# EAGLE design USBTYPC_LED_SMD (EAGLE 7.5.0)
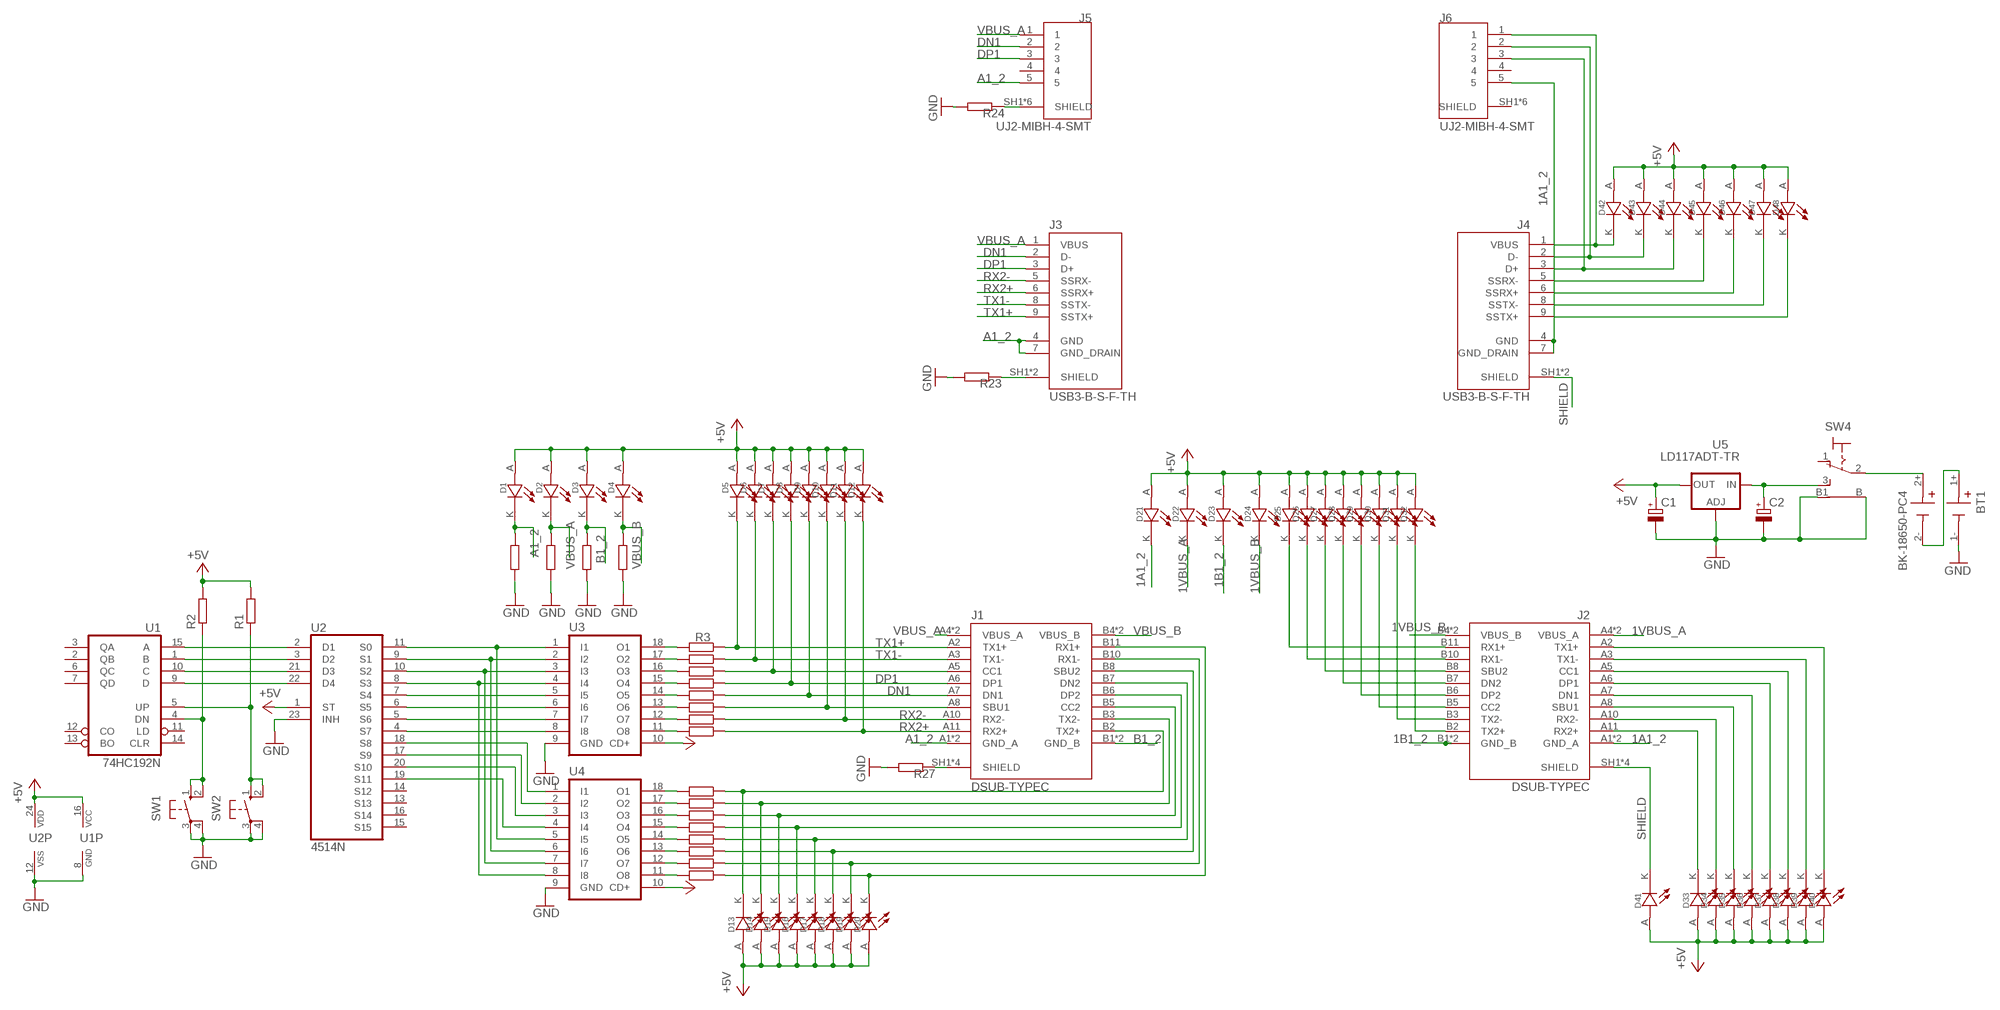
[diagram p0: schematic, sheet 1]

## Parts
BT1  BK-18650-PC4  [BAT_BK-18650-PC4]
C1  CPOL-EUSMCD  [SMC_D]
C2  CPOL-EUSMCD  [SMC_D]
D1  597-6401-607F  [LED_597-6401-607F]
D2  597-6401-607F  [LED_597-6401-607F]
D3  597-6401-607F  [LED_597-6401-607F]
D4  597-6401-607F  [LED_597-6401-607F]
D5  597-6401-607F  [LED_597-6401-607F]
D6  597-6401-607F  [LED_597-6401-607F]
D7  597-6401-607F  [LED_597-6401-607F]
D8  597-6401-607F  [LED_597-6401-607F]
D9  597-6401-607F  [LED_597-6401-607F]
D10  597-6401-607F  [LED_597-6401-607F]
D11  597-6401-607F  [LED_597-6401-607F]
D12  597-6401-607F  [LED_597-6401-607F]
D13  597-6401-607F  [LED_597-6401-607F]
D14  597-6401-607F  [LED_597-6401-607F]
D15  597-6401-607F  [LED_597-6401-607F]
D16  597-6401-607F  [LED_597-6401-607F]
D17  597-6401-607F  [LED_597-6401-607F]
D18  597-6401-607F  [LED_597-6401-607F]
D19  597-6401-607F  [LED_597-6401-607F]
D20  597-6401-607F  [LED_597-6401-607F]
D21  597-6401-607F  [LED_597-6401-607F]
D22  597-6401-607F  [LED_597-6401-607F]
D23  597-6401-607F  [LED_597-6401-607F]
D24  597-6401-607F  [LED_597-6401-607F]
D25  597-6401-607F  [LED_597-6401-607F]
D26  597-6401-607F  [LED_597-6401-607F]
D27  597-6401-607F  [LED_597-6401-607F]
D28  597-6401-607F  [LED_597-6401-607F]
D29  597-6401-607F  [LED_597-6401-607F]
D30  597-6401-607F  [LED_597-6401-607F]
D31  597-6401-607F  [LED_597-6401-607F]
D32  597-6401-607F  [LED_597-6401-607F]
D33  597-6401-607F  [LED_597-6401-607F]
D34  597-6401-607F  [LED_597-6401-607F]
D35  597-6401-607F  [LED_597-6401-607F]
D36  597-6401-607F  [LED_597-6401-607F]
D37  597-6401-607F  [LED_597-6401-607F]
D38  597-6401-607F  [LED_597-6401-607F]
D39  597-6401-607F  [LED_597-6401-607F]
D40  597-6401-607F  [LED_597-6401-607F]
D41  597-6401-607F  [LED_597-6401-607F]
D42  597-6401-607F  [LED_597-6401-607F]
D43  597-6401-607F  [LED_597-6401-607F]
D44  597-6401-607F  [LED_597-6401-607F]
D45  597-6401-607F  [LED_597-6401-607F]
D46  597-6401-607F  [LED_597-6401-607F]
D47  597-6401-607F  [LED_597-6401-607F]
D48  597-6401-607F  [LED_597-6401-607F]
J1  DSUB-TYPEC  2345986-1  [TE_2345986-1]
J2  DSUB-TYPEC  2345986-1  [TE_2345986-1]
J3  USB3-B-S-F-TH  [SAMTEC_USB3-B-S-F-TH]
J4  USB3-B-S-F-TH  [SAMTEC_USB3-B-S-F-TH]
J5  UJ2-MIBH-4-SMT  [CUI_UJ2-MIBH-4-SMT]
J6  UJ2-MIBH-4-SMT  [CUI_UJ2-MIBH-4-SMT]
R1  R-EU_R1206  [R1206]
R2  R-EU_R1206  [R1206]
R3  R-EU_R1206  [R1206]
R4  R-EU_R1206  [R1206]
R5  R-EU_R1206  [R1206]
R6  R-EU_R1206  [R1206]
R7  R-EU_R1206  [R1206]
R8  R-EU_R1206  [R1206]
R9  R-EU_R1206  [R1206]
R10  R-EU_R1206  [R1206]
R11  R-EU_R1206  [R1206]
R12  R-EU_R1206  [R1206]
R13  R-EU_R1206  [R1206]
R14  R-EU_R1206  [R1206]
R15  R-EU_R1206  [R1206]
R16  R-EU_R1206  [R1206]
R17  R-EU_R1206  [R1206]
R18  R-EU_R1206  [R1206]
R19  R-EU_R1206  [R1206]
R20  R-EU_R1206  [R1206]
R21  R-EU_R1206  [R1206]
R22  R-EU_R1206  [R1206]
R23  R-EU_R1206  [R1206]
R24  R-EU_R1206  [R1206]
R27  R-EU_R1206  [R1206]
SW1  10-XX  [B3F-10XX]
SW2  10-XX  [B3F-10XX]
SW4  9070-1W  [9070-1W]
U1  74HC192N  [DIL16]
U2  4514N  [DIL24-6]
U3  ULN2803A  [DIL18]
U4  ULN2803A  [DIL18]
U5  LD117ADT-TR  [DPACK]

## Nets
1A1_2: D21.K(CATHODE) J2.A1(GND_A) J2.A12(GND_A) J4.4(GND) J4.7(GND_DRAIN) J6.5
1B1_2: D23.K(CATHODE) J2.B1(GND_B) J2.B12(GND_B)
1VBUS_A: D22.K(CATHODE) J2.A4(VBUS_A) J2.A9(VBUS_A)
1VBUS_B: D24.K(CATHODE) J2.B4(VBUS_B) J2.B9(VBUS_B)
+5V: C1.+ D1.A(ANODE) D2.A(ANODE) D3.A(ANODE) D4.A(ANODE) D5.A(ANODE) D6.A(ANODE) D7.A(ANODE) D8.A(ANODE) D9.A(ANODE) D10.A(ANODE) D11.A(ANODE) D12.A(ANODE) D13.A(ANODE) D14.A(ANODE) D15.A(ANODE) D16.A(ANODE) D17.A(ANODE) D18.A(ANODE) D19.A(ANODE) D20.A(ANODE) D21.A(ANODE) D22.A(ANODE) D23.A(ANODE) D24.A(ANODE) D25.A(ANODE) D26.A(ANODE) D27.A(ANODE) D28.A(ANODE) D29.A(ANODE) D30.A(ANODE) D31.A(ANODE) D32.A(ANODE) D33.A(ANODE) D34.A(ANODE) D35.A(ANODE) D36.A(ANODE) D37.A(ANODE) D38.A(ANODE) D39.A(ANODE) D40.A(ANODE) D41.A(ANODE) D42.A(ANODE) D43.A(ANODE) D44.A(ANODE) D45.A(ANODE) D46.A(ANODE) D47.A(ANODE) D48.A(ANODE) R1.2 R2.2 U1.16(VCC) U2.1(ST) U2.24(VDD) U3.10(CD+) U4.10(CD+) U5.4(OUT)
A1_2: D1.K(CATHODE) J1.A1(GND_A) J1.A12(GND_A) J3.4(GND) J3.7(GND_DRAIN) J5.5 R19.1
B1_2: D3.K(CATHODE) J1.B1(GND_B) J1.B12(GND_B) R21.1
DN1: D9.K(CATHODE) J1.A7(DN1) J3.2(D-) J5.2 R7.1
DP1: D8.K(CATHODE) J1.A6(DP1) J3.3(D+) J5.3 R6.1
GND: BT1.1- C1.- C2.- R19.2 R20.2 R21.2 R22.2 R23.2 R24.2 R27.2 SW1.3(P) SW1.4(P1) SW2.3(P) SW2.4(P1) SW4.B SW4.B1 U1.8(GND) U2.12(VSS) U2.23(INH) U3.9(GND) U4.9(GND) U5.1(ADJ)
N$1: U1.15(A) U2.2(D1)
N$2: U1.1(B) U2.3(D2)
N$3: U1.10(C) U2.21(D3)
N$4: U1.9(D) U2.22(D4)
N$5: R3.2 U3.18(O1)
N$6: R4.2 U3.17(O2)
N$7: R1.1 SW2.1(S) SW2.2(S1) U1.5(UP)
N$8: U2.10(S2) U3.3(I3) U4.7(I7)
N$9: R2.1 SW1.1(S) SW1.2(S1) U1.4(DN)
N$10: U2.8(S3) U3.4(I4) U4.8(I8)
N$11: U2.7(S4) U3.5(I5)
N$12: U2.6(S5) U3.6(I6)
N$13: U2.5(S6) U3.7(I7)
N$14: U2.4(S7) U3.8(I8)
N$15: U2.19(S11) U4.4(I4)
N$16: U2.18(S8) U4.1(I1)
N$17: U2.17(S9) U4.2(I2)
N$18: U2.20(S10) U4.3(I3)
N$19: U2.11(S0) U3.1(I1) U4.5(I5)
N$20: U2.9(S1) U3.2(I2) U4.6(I6)
N$21: R5.2 U3.16(O3)
N$22: R6.2 U3.15(O4)
N$23: R7.2 U3.14(O5)
N$24: R8.2 U3.13(O6)
N$25: R9.2 U3.12(O7)
N$26: R10.2 U3.11(O8)
N$27: R11.2 U4.18(O1)
N$28: R12.2 U4.17(O2)
N$29: R13.2 U4.16(O3)
N$30: R14.2 U4.15(O4)
N$31: R15.2 U4.14(O5)
N$32: R16.2 U4.13(O6)
N$33: R17.2 U4.12(O7)
N$34: R18.2 U4.11(O8)
N$35: J5.SH1(SHIELD) J5.SH2(SHIELD) J5.SH3(SHIELD) J5.SH4(SHIELD) J5.SH5(SHIELD) J5.SH6(SHIELD) R24.1
N$36: D42.K(CATHODE) J4.1(VBUS) J6.1
N$37: D25.K(CATHODE) J2.B11(RX1+)
N$38: D7.K(CATHODE) J1.A5(CC1) R5.1
N$39: D43.K(CATHODE) J4.2(D-) J6.2
N$40: D44.K(CATHODE) J4.3(D+) J6.3
N$41: D10.K(CATHODE) J1.A8(SBU1) R8.1
N$42: D45.K(CATHODE) J4.5(SSRX-)
N$43: D46.K(CATHODE) J4.6(SSRX+)
N$44: D26.K(CATHODE) J2.B10(RX1-)
N$45: D13.K(CATHODE) J1.B2(TX2+) R11.1
N$46: D14.K(CATHODE) J1.B3(TX2-) R12.1
N$47: D15.K(CATHODE) J1.B5(CC2) R13.1
N$48: D16.K(CATHODE) J1.B6(DP2) R14.1
N$49: D17.K(CATHODE) J1.B7(DN2) R15.1
N$50: D18.K(CATHODE) J1.B8(SBU2) R16.1
N$51: D19.K(CATHODE) J1.B10(RX1-) R17.1
N$52: D20.K(CATHODE) J1.B11(RX1+) R18.1
N$53: D27.K(CATHODE) J2.B8(SBU2)
N$54: D28.K(CATHODE) J2.B7(DN2)
N$55: D29.K(CATHODE) J2.B6(DP2)
N$56: D30.K(CATHODE) J2.B5(CC2)
N$57: D31.K(CATHODE) J2.B3(TX2-)
N$58: D32.K(CATHODE) J2.B2(TX2+)
N$59: D33.K(CATHODE) J2.A11(RX2+)
N$60: D34.K(CATHODE) J2.A10(RX2-)
N$61: D35.K(CATHODE) J2.A8(SBU1)
N$62: D36.K(CATHODE) J2.A7(DN1)
N$63: D37.K(CATHODE) J2.A6(DP1)
N$64: D38.K(CATHODE) J2.A5(CC1)
N$65: D39.K(CATHODE) J2.A3(TX1-)
N$66: D40.K(CATHODE) J2.A2(TX1+)
N$67: J3.SH1(SHIELD) J3.SH2(SHIELD) R23.1
N$68: D47.K(CATHODE) J4.8(SSTX-)
N$69: D48.K(CATHODE) J4.9(SSTX+)
N$75: J1.SH1(SHIELD) J1.SH2(SHIELD) J1.SH3(SHIELD) J1.SH4(SHIELD) R27.1
N$120: BT1.2+ SW4.2(P)
N$121: C2.+ SW4.3(S) U5.3(IN)
N$122: BT1.1+ BT1.2-
RX2+: D12.K(CATHODE) J1.A11(RX2+) J3.6(SSRX+) R10.1
RX2-: D11.K(CATHODE) J1.A10(RX2-) J3.5(SSRX-) R9.1
SHIELD: D41.K(CATHODE) J2.SH1(SHIELD) J2.SH2(SHIELD) J2.SH3(SHIELD) J2.SH4(SHIELD) J4.SH1(SHIELD) J4.SH2(SHIELD)
TX1+: D5.K(CATHODE) J1.A2(TX1+) J3.9(SSTX+) R3.1
TX1-: D6.K(CATHODE) J1.A3(TX1-) J3.8(SSTX-) R4.1
VBUS_A: D2.K(CATHODE) J1.A4(VBUS_A) J1.A9(VBUS_A) J3.1(VBUS) J5.1 R20.1
VBUS_B: D4.K(CATHODE) J1.B4(VBUS_B) J1.B9(VBUS_B) R22.1
Unconnected: J5.4 J6.4 J6.SH1(SHIELD) J6.SH2(SHIELD) J6.SH3(SHIELD) J6.SH4(SHIELD) J6.SH5(SHIELD) J6.SH6(SHIELD) SW4.1(O) U1.2(QB) U1.3(QA) U1.6(QC) U1.7(QD) U1.11(LD) U1.12(CO) U1.13(BO) U1.14(CLR) U2.13(S13) U2.14(S12) U2.15(S15) U2.16(S14)

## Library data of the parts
BT1 = BK-18650-PC4:BK-18650-PC4: Battery Holder (Open) 18650 2 Cell PC Pin Check availability; AVAILABILITY: In Stock; CHECK_PRICES: https://www.snapeda.com/parts/BK-18650-PC4/Memory+Protection+Devices/view-part/?ref=eda; DESCRIPTION: Battery Holder (Open) 18650 2 Cell PC Pin; MF: MPD (Memory Protection Devices); MP: BK-18650-PC4; PACKAGE: None; PRICE: None; SNAPEDA_LINK: https://www.snapeda.com/parts/BK-18650-PC4/Memory+Protection+Devices/view-part/?ref=snap
C1 C2 = rcl:CPOL-EU: POLARIZED CAPACITOR, European symbol
D1-D48 = LED1206:597-6401-607F: Check availability; AVAILABILITY: In Stock; CHECK_PRICES: https://www.snapeda.com/parts/597-6401-607F/Dialight/view-part/?ref=eda; DESCRIPTION: Indicators; Reverse Mount; LED; SMD; Yellow; Right Angle; 25 mA | Dialight 597-6401-607F; MF: Dialight; MP: 597-6401-607F; PACKAGE: 1206 Dialight; PRICE: None; PURCHASE-URL: https://www.snapeda.com/api/url_track_click_mouser/?unipart_id=301068&manufacturer=Dialight&part_name=597-6401-607F&search_term=smd led; SNAPEDA_LINK: https://www.snapeda.com/parts/597-6401-607F/Dialight/view-part/?ref=snap
J1 J2 = USB_C:2345986-1: Check availability; AVAILABILITY: In Stock; CHECK_PRICES: https://www.snapeda.com/parts/2345986-1/TE+Connectivity/view-part/?ref=eda; DESCRIPTION: USB TYPE C 3.1 TOP MOUNT DUAL SMT 1.63CH; MF: TE Connectivity; MP: 2345986-1; PACKAGE: None; PRICE: None; PURCHASE-URL: https://www.snapeda.com/api/url_track_click_mouser/?unipart_id=9344621&manufacturer=TE Connectivity&part_name=2345986-1&search_term=usb type c; SNAPEDA_LINK: https://www.snapeda.com/parts/2345986-1/TE+Connectivity/view-part/?ref=snap
J3 J4 = USB3-B-S-F-TH:USB3-B-S-F-TH: Check availability; AVAILABILITY: Not in stock; CHECK_PRICES: https://www.snapeda.com/parts/USB3-B-S-F-TH/Samtec/view-part/?ref=eda; DESCRIPTION: Conn USB 3.0 Type B PL 4 POS Solder RA Thru-Hole 4 Terminal 1 Port; MF: Samtec; MP: USB3-B-S-F-TH; PACKAGE: None; PRICE: None; PURCHASE-URL: https://www.snapeda.com/api/url_track_click_mouser/?unipart_id=378053&manufacturer=Samtec&part_name=USB3-B-S-F-TH&search_term=usb 3.0; SNAPEDA_LINK: https://www.snapeda.com/parts/USB3-B-S-F-TH/Samtec/view-part/?ref=snap
J5 J6 = UJ2-MIBH-4-SMTE EAGLE:UJ2-MIBH-4-SMT: Micro B, USB 2.0, 1.8 A, Right Angle, Surface Mount (SMT), USB Receptacle Check availability; AVAILABILITY: Not in stock; CHECK_PRICES: https://www.snapeda.com/parts/UJ2-MIBH-4-SMT/Same+Sky/view-part/?ref=eda; DESCRIPTION: Micro B, USB 2.0, 480 Mbps, 30 Vac, 1.8 A, Right Angle, Surface Mount, USB Receptacle; MF: Same Sky; MP: UJ2-MIBH-4-SMT; PACKAGE: None; PRICE: None; PURCHASE-URL: https://www.snapeda.com/api/url_track_click_mouser/?unipart_id=4299825&manufacturer=Same Sky&part_name=UJ2-MIBH-4-SMT&search_term=usb micro; SNAPEDA_LINK: https://www.snapeda.com/parts/UJ2-MIBH-4-SMT/Same+Sky/view-part/?ref=snap
R1-R24 R27 = rcl:R-EU_: RESISTOR, European symbol
SW1 SW2 = switch-omron:10-XX: OMRON SWITCH; MPN: B3F-1000; OC_FARNELL: 176432; OC_NEWARK: 36M3542
SW4 = switch:9070-1W: TOGGLE SWITCH Marquardt
U1 = 74xx-eu:74*192: Synchronous 4-bit UP/DOWN COUNTER
U2 = 45xx:4514: 4-bit latch 4-16 line DECODER
U3 U4 = uln-udn:ULN2803A: DRIVER ARRAY
U5 = v-reg:LD117A?*: Low drop fixed and adjustable positive voltage regulators 1 A Source: http://www.st.com/stonline/products/literature/ds/7194/ld1117axx.pdf

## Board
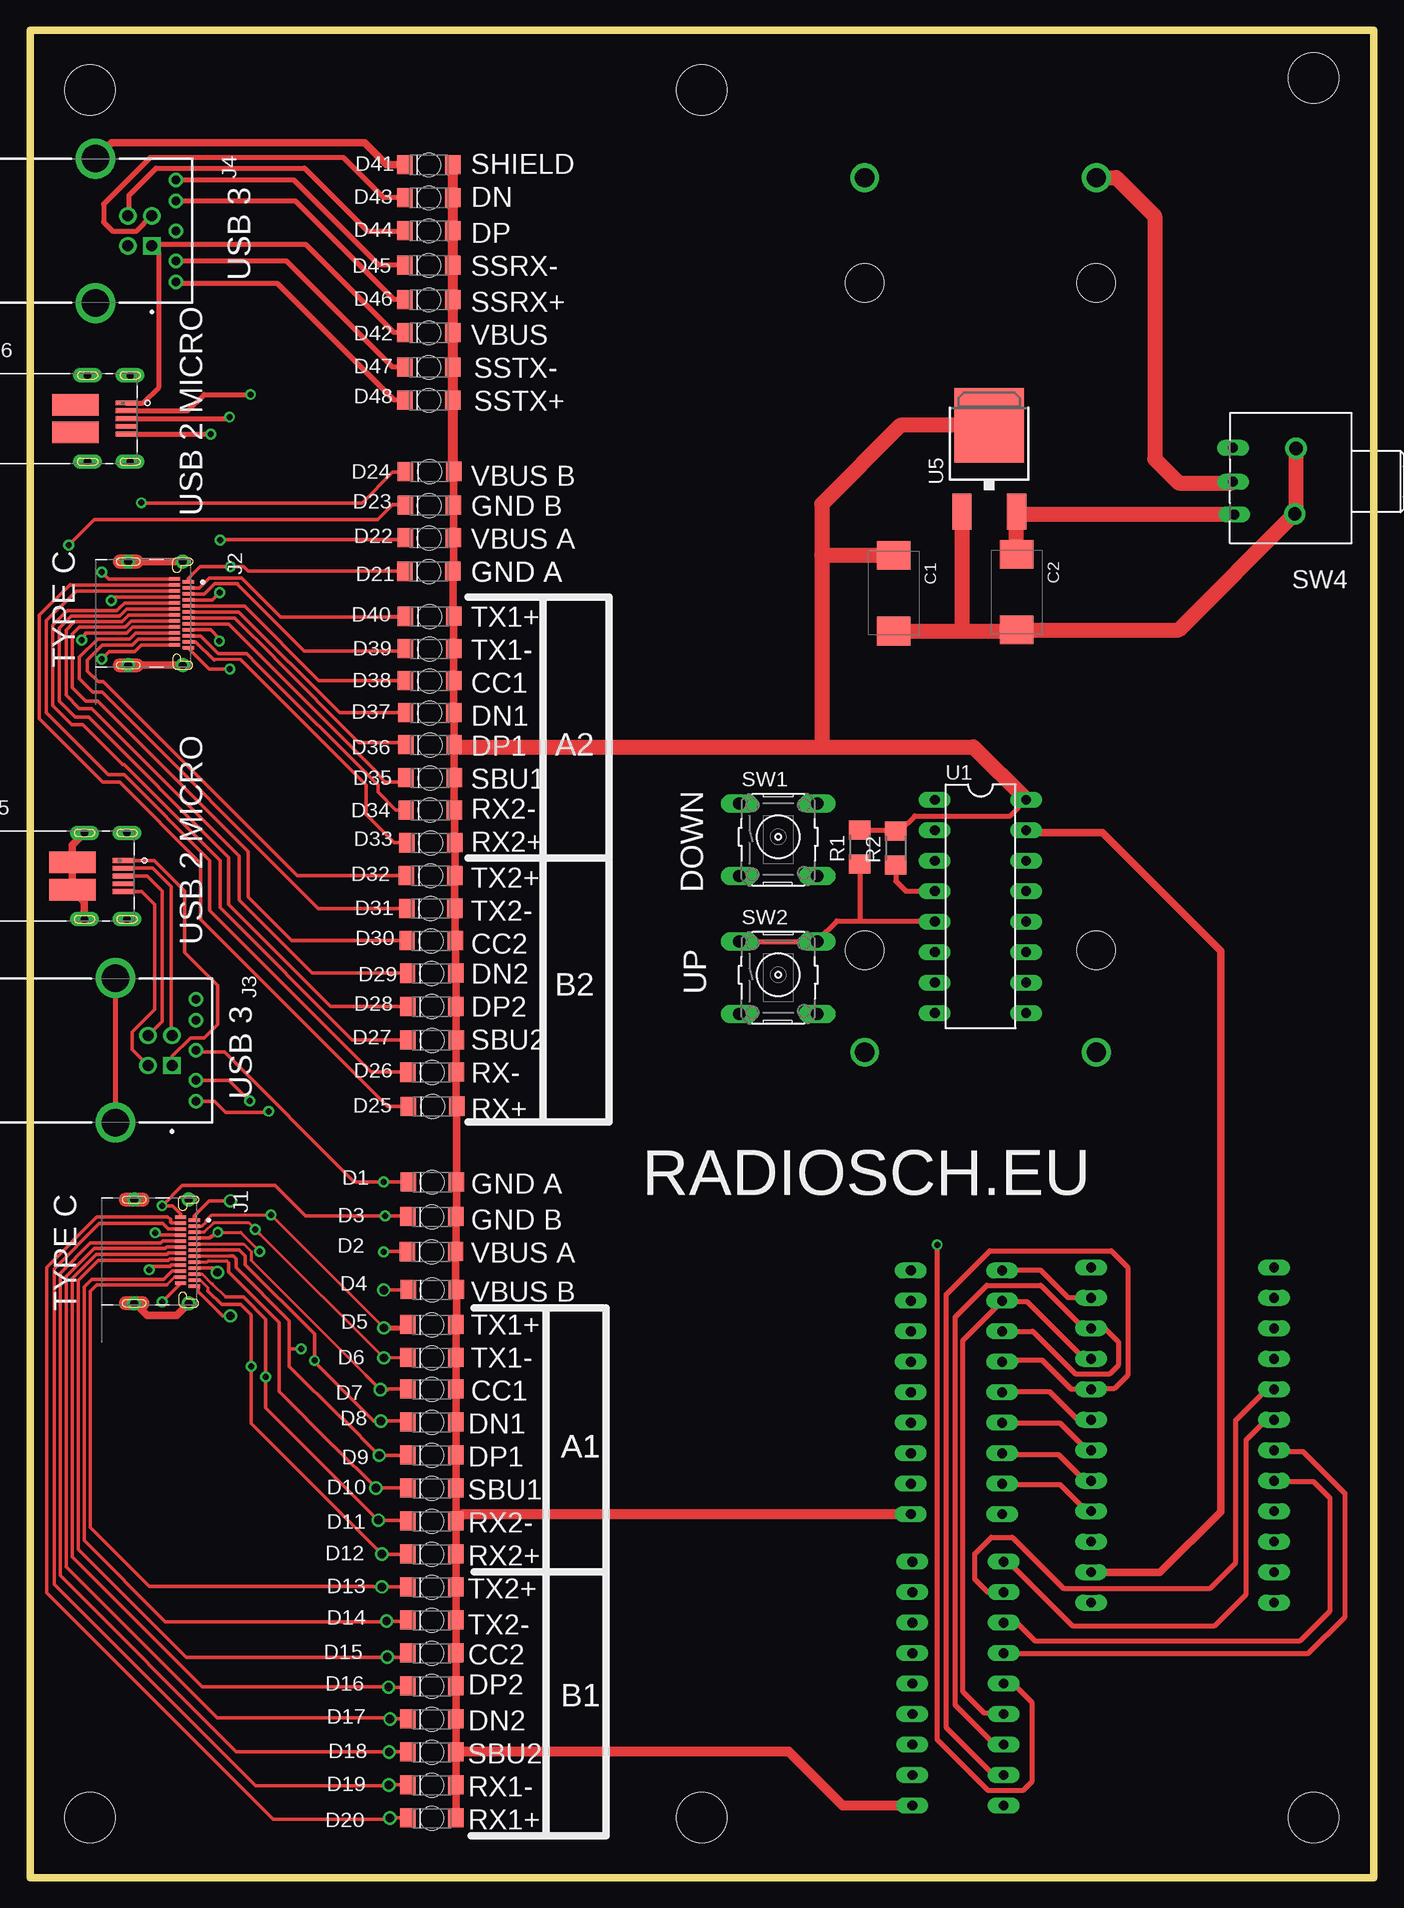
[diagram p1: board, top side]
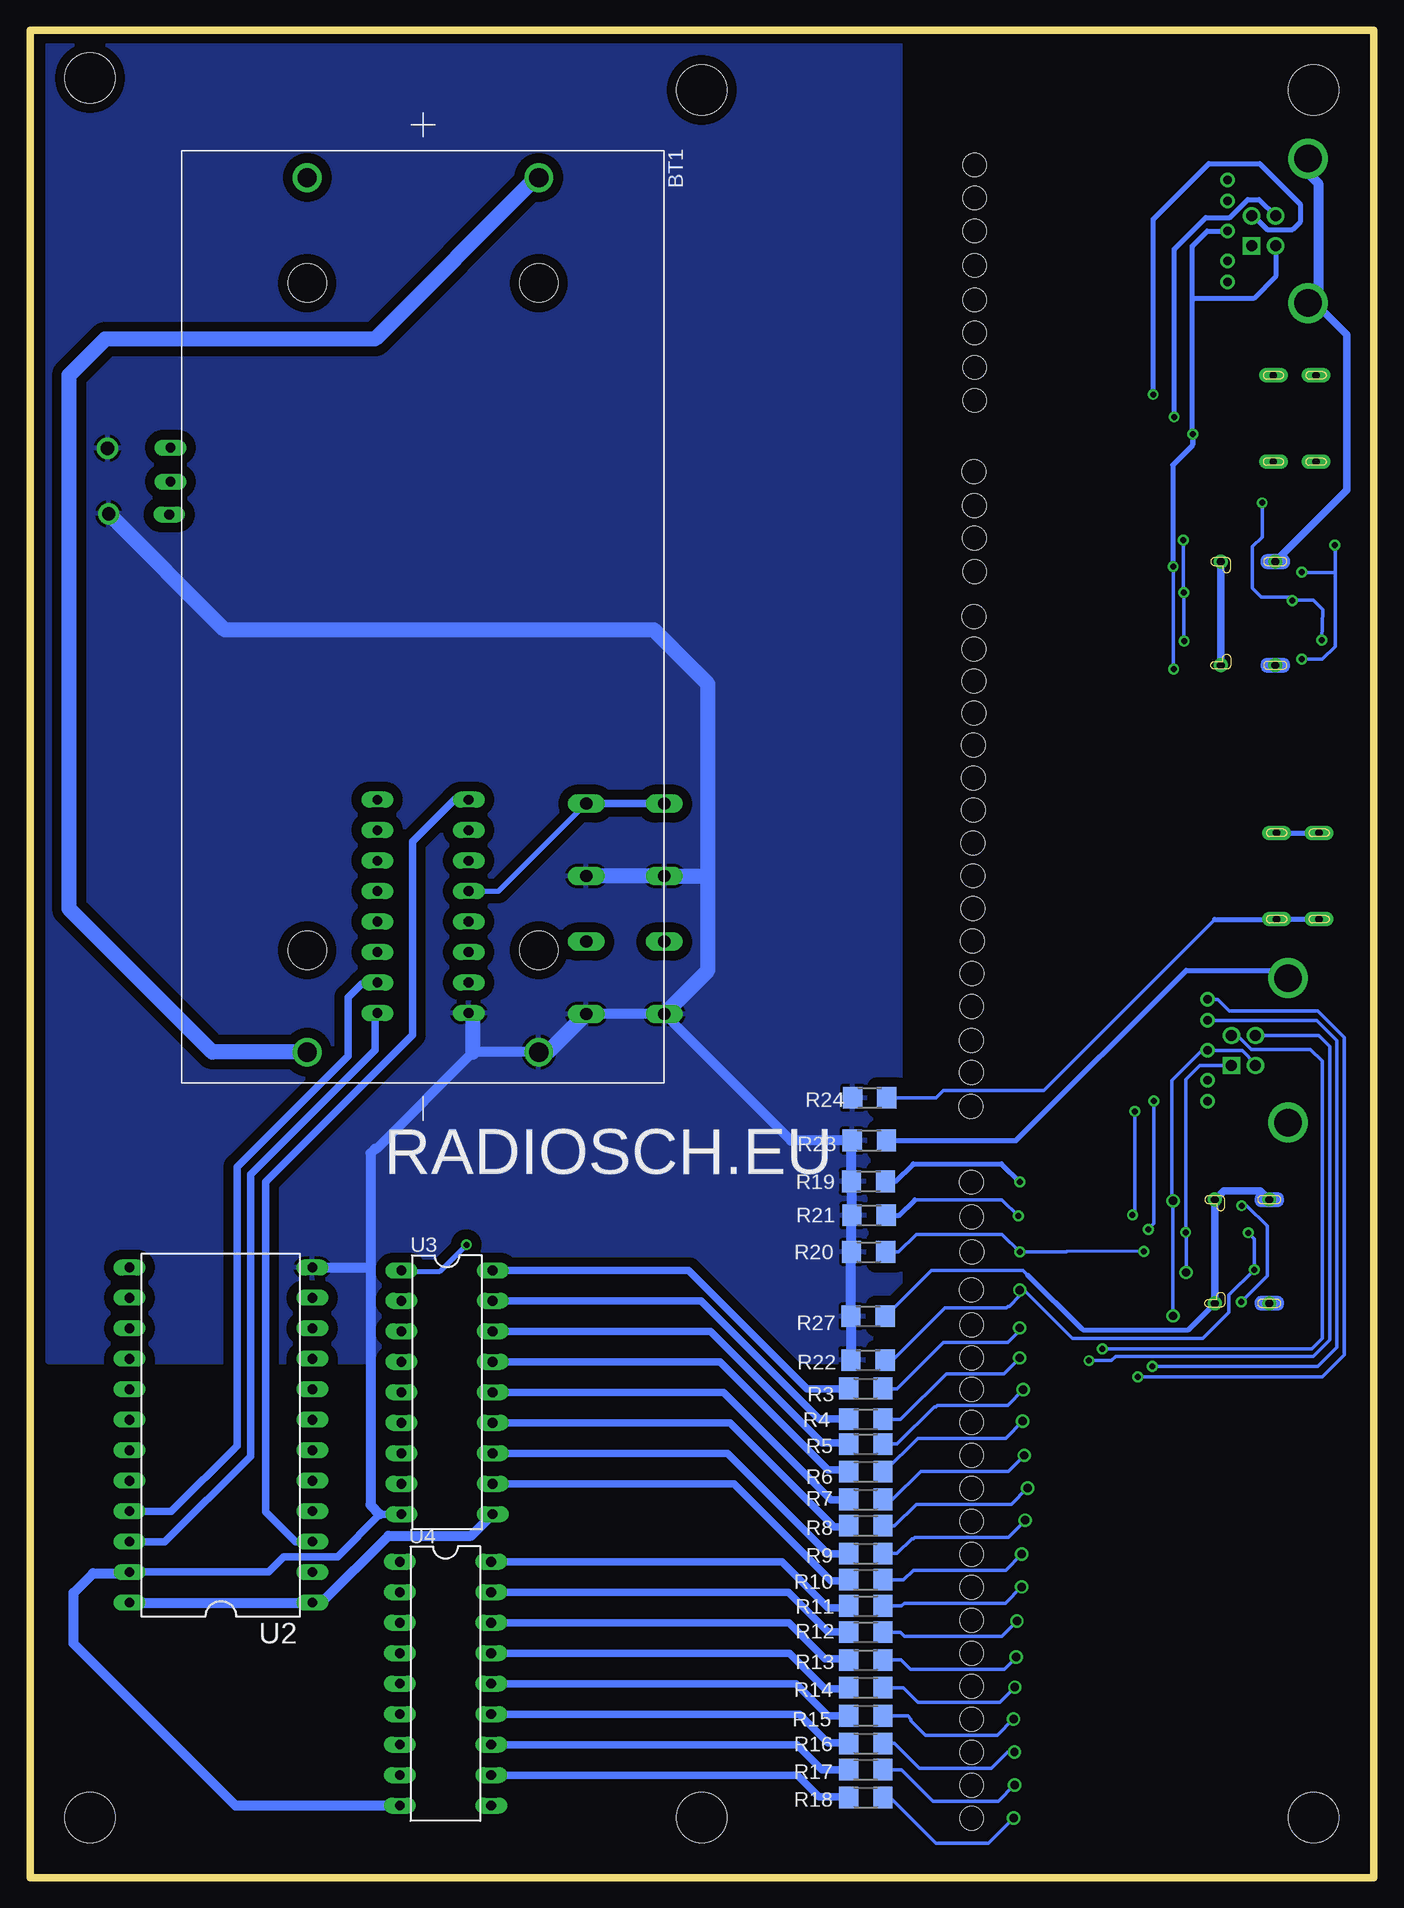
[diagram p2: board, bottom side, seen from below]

Size 112 x 154 mm. Coordinates in mm from the lower left corner, seen from the top.
Outline: 0,0 0,154 112,154 112,0 0,0
Copper layers (1*16): Top 0.035mm / dielectric 1.5mm / Bottom 0.035mm
Design rules "default *": minimum track width 10mil, minimum drill 18mil, track to track 5mil, track to pad 5mil, pad to pad 6mil, via to via 6mil, smd to smd 6mil, copper to edge 6mil, drill to drill 8mil, minimum pad ring 10mil, minimum via ring 8mil, stop-mask expansion 4mil, vias tented up to drill 0mil, thermal gap 10mil
Holes 4.2 mm at 5,5 107,5 56,5 5,149 107,150 56,149

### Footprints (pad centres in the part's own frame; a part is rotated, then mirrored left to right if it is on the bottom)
BAT_BK-18650-PC4 = drill 1.6: 1+ -36.6,9.65; 1- 36.3,9.65; 2+ -36.6,-9.65; 2- 36.3,-9.65 | hole 3.2: -27.81,-9.65; -27.81,9.65; 27.81,-9.65; 27.81,9.65
SMC_D = smd 2.4 x 2.8: + -3.15,0; - 3.15,0
LED_597-6401-607F = smd 1.284 x 1.59: A 2.017,0.033; K -2.01,0.026 | hole 1.98: 0,0
TE_2345986-1 = smd 0.3 x 0.95: A1 -2.62,3.765; A2 -2.12,3.765; A3 -1.62,3.765; A4 -1.12,3.765; A5 -0.62,3.765; A6 -0.12,3.765; A7 0.38,3.765; A8 0.88,3.765; A9 1.38,3.765; A10 1.88,3.765; A11 2.38,3.765; A12 2.88,3.765; B1 2.63,2.625; B2 2.13,2.625; B3 1.63,2.625; B4 1.13,2.625; B5 0.63,2.625; B6 0.13,2.625; B7 -0.37,2.625; B8 -0.87,2.625; B9 -1.37,2.625; B10 -1.87,2.625; B11 -2.37,2.625; B12 -2.87,2.625 | drill 0.65 pad 1.14: SH1 -4.32,3.3; SH2 4.32,3.3; SH3 -4.32,-1.25; SH4 4.32,-1.25
SAMTEC_USB3-B-S-F-TH = drill 0.92 square: 1 1.25,4.71 | drill 0.92: 2 -1.25,4.71; 3 -1.25,2.71; 4 1.25,2.71 | drill 0.7: 5 -4.25,6.71; 6 -2.5,6.71; 7 0,6.71; 8 2.5,6.71; 9 4.25,6.71 | drill 2.3: SH1 -6.02,0; SH2 6.02,0
CUI_UJ2-MIBH-4-SMT = smd 1.7 x 0.4: 1 0,0.03; 2 0,-0.62; 3 0,-1.27; 4 0,-1.92; 5 0,-2.57 | drill 0.6 pad 1.2 long: SH1 -3.2,2.33; SH2 0.35,2.33; SH5 -3.2,-4.87; SH6 0.35,-4.87 | smd 3.9 x 1.8: SH3 -4.2,-0.12; SH4 -4.2,-2.42
R1206 = smd 1.6 x 1.803: 1 -1.422,0; 2 1.422,0
B3F-10XX = drill 1.016 long: 1 -3.251,2.761; 2 3.251,2.761; 3 -3.251,-3.261; 4 3.251,-3.261
9070-1W = drill 0.813 long: 1 5.08,-2.835; 2 5.08,0; 3 4.98,2.735 | drill 1.118 pad 1.778: B -0.161,-2.794; B1 -0.061,2.667
DIL16 = drill 0.813 long: 1 -8.89,-3.81; 2 -6.35,-3.81; 3 -3.81,-3.81; 4 -1.27,-3.81; 5 1.27,-3.81; 6 3.81,-3.81; 7 6.35,-3.81; 8 8.89,-3.81; 9 8.89,3.81; 10 6.35,3.81; 11 3.81,3.81; 12 1.27,3.81; 13 -1.27,3.81; 14 -3.81,3.81; 15 -6.35,3.81; 16 -8.89,3.81
DIL24-6 = drill 0.813 long: 1 -13.97,-7.62; 2 -11.43,-7.62; 3 -8.89,-7.62; 4 -6.35,-7.62; 5 -3.81,-7.62; 6 -1.27,-7.62; 7 1.27,-7.62; 8 3.81,-7.62; 9 6.35,-7.62; 10 8.89,-7.62; 11 11.43,-7.62; 12 13.97,-7.62; 13 13.97,7.62; 14 11.43,7.62; 15 8.89,7.62; 16 6.35,7.62; 17 3.81,7.62; 18 1.27,7.62; 19 -1.27,7.62; 20 -3.81,7.62; 21 -6.35,7.62; 22 -8.89,7.62; 23 -11.43,7.62; 24 -13.97,7.62
DIL18 = drill 0.813 long: 1 -10.16,-3.81; 2 -7.62,-3.81; 3 -5.08,-3.81; 4 -2.54,-3.81; 5 0,-3.81; 6 2.54,-3.81; 7 5.08,-3.81; 8 7.62,-3.81; 9 10.16,-3.81; 10 10.16,3.81; 11 7.62,3.81; 12 5.08,3.81; 13 2.54,3.81; 14 0,3.81; 15 -2.54,3.81; 16 -5.08,3.81; 17 -7.62,3.81; 18 -10.16,3.81
DPACK = smd 1.6 x 3: 1 -2.28,-4.8; 3 2.28,-4.8 | smd 5.8 x 6.2: 4 0,2.38

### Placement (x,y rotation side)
BT1  79.23,105.1 270 bottom
C1  72,107.06 270 top
C2  82.25,107.14 270 top
D1  33.54,57.96 0 top
D2  33.46,52.14 0 top
D3  33.5,55.07 0 top
D4  33.54,48.99 0 top
D5  33.5,46.06 0 top
D6  33.5,43.31 0 top
D7  33.5,40.69 0 top
D8  33.5,37.94 0 top
D9  33.5,35.19 0 top
D10  33.5,32.44 0 top
D11  33.5,29.69 0 top
D12  33.5,26.94 0 top
D13  33.5,24.19 0 top
D14  33.5,21.44 0 top
D15  33.5,18.69 0 top
D16  33.5,15.94 0 top
D17  33.5,13.19 0 top
D18  33.5,10.44 0 top
D19  33.5,7.69 0 top
D20  33.5,4.94 0 top
D21  33.25,108.85 0 top
D22  33.29,111.65 0 top
D23  33.29,114.36 0 top
D24  33.31,117.17 0 top
D25  33.56,64.26 0 top
D26  33.51,67.1 0 top
D27  33.51,69.79 0 top
D28  33.5,72.59 0 top
D29  33.49,75.35 0 top
D30  33.45,78.06 0 top
D31  33.41,80.76 0 top
D32  33.4,83.5 0 top
D33  33.41,86.22 0 top
D34  33.36,88.96 0 top
D35  33.35,91.65 0 top
D36  33.34,94.4 0 top
D37  33.33,97.07 0 top
D38  33.31,99.74 0 top
D39  33.31,102.4 0 top
D40  33.31,105.1 0 top
D41  33.25,142.75 0 top
D42  33.25,128.75 0 top
D43  33.25,140 0 top
D44  33.25,137.25 0 top
D45  33.25,134.38 0 top
D46  33.25,131.5 0 top
D47  33.25,125.88 0 top
D48  33.25,123.12 0 top
J1  9.94,52.19 270 top
J2  9.44,105.37 270 top
J3  7.13,68.95 270 top
J4  5.45,137.26 270 top
J5  7.74,84.75 0 top
J6  8,122.88 0 top
R1  69.17,85.89 90 top
R2  72.17,85.81 90 top
R3  42.33,40.77 180 bottom
R4  42.33,38.21 180 bottom
R5  42.33,36.14 180 bottom
R6  42.33,33.83 180 bottom
R7  42.33,31.52 180 bottom
R8  42.33,29.32 180 bottom
R9  42.33,27.01 180 bottom
R10  42.33,24.83 180 bottom
R11  42.33,22.64 180 bottom
R12  42.33,20.45 180 bottom
R13  42.33,18.14 180 bottom
R14  42.33,15.83 180 bottom
R15  42.33,13.48 180 bottom
R16  42.33,11.17 180 bottom
R17  42.33,8.99 180 bottom
R18  42.33,6.67 180 bottom
R19  42.1,58.02 180 bottom
R20  42.09,52.14 180 bottom
R21  42.05,55.2 180 bottom
R22  42.14,43.14 180 bottom
R23  42.04,61.44 180 bottom
R24  42,65 180 bottom
R27  42.13,46.78 180 bottom
SW1  62.38,86.75 0 top
SW2  62.38,75.25 0 top
SW4  105.38,116.34 180 top
U1  79.24,80.95 270 top
U2  96.08,36.88 90 bottom
U3  77.24,40.44 270 bottom
U4  77.36,16.16 270 bottom
U5  79.97,118.67 0 top

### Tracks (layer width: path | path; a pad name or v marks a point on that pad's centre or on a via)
1A1_2  (via drill 0.5)
  Top 0.305: J2.A1 13.2,108.29 14.18,109.26 v16.7,109.26 | v16.67,100.74 14.96,100.74 J2.A12 | D21.K 18.19,108.88 17.81,109.26 v16.7,109.26 | v16.7,109.26
  Top 0.406: J6.5 v15.06,120.31
  Bottom 0.305: v16.7,109.26 16.7,100.77 v16.67,100.74
  Bottom 0.406: 15.12,131.5 15.12,120.38 v15.06,120.31 | 15.12,131.5 15.12,136 13.88,137.25 J4.7 | J4.4 8.16,133.46 10,131.62 15,131.62 15.12,131.5 | v15.06,120.31 15.06,119.44 15.12,119.38 | 15.12,119.38 16.75,117.75 16.75,109.31 v16.7,109.26 | v15.06,120.31 15.12,119.38
1B1_2  (via drill 0.5)
  Top 0.305: J2.B12 6.58,108.24 v5.99,108.82 | J2.B1 9.28,102.74 8.72,102.17 6.6,102.17 v5.99,101.56 | v3.24,111.05 5.37,113.17 28.98,113.17 30.23,114.43 31.24,114.43 D23.K
  Bottom 0.305: v5.99,101.56 4.27,101.56 3.2,102.62 3.2,108.65 | 3.2,108.65 3.2,111.01 v3.24,111.05 | v5.99,108.82 5.95,108.79 3.34,108.79 3.2,108.65
1VBUS_A  (via drill 0.5)
  Top 0.305: J2.A4 15.21,106.49 v15.82,107.1 | v15.79,103.07 15.79,103.29 15.07,104.01 13.23,104.01 J2.A9 | v15.84,111.47 15.89,111.52 31.13,111.52 D22.K
  Bottom 0.305: v15.79,103.07 15.82,103.1 v15.82,107.1 15.84,107.12 v15.84,111.47
1VBUS_B  (via drill 0.5)
  Top 0.305: J2.B9 7.08,106.74 v6.78,106.44 | J2.B4 10.86,104.24 10.83,104.21 8.55,104.21 8.08,103.74 4.65,103.74 v4.32,103.16 | v9.29,114.59 9.3,114.57 27.67,114.57 30.23,117.13 31.23,117.13 D24.K
  Bottom 0.305: v4.32,103.16 4.23,105.67 5.04,106.49 6.73,106.49 v6.78,106.44 7.08,106.74 9.35,106.74 10.09,107.48 10.09,110.92 9.29,111.72 v9.29,114.59
+5V
  Top 0.406: R1.2 72.09,87.31 R2.2 72.48,87.23 73.75,88.5 81.71,88.5 U1.16 | D33.A 35.43,93.93 35.75,94.25
  Top 0.61: 35.27,117.27 D24.A 35.33,114.42 D23.A D22.A 35.3,108.92 D21.A 35.27,105.19 D40.A D39.A D38.A D37.A 35.34,94.44 D36.A 35.35,91.69 D35.A 35.37,89.01 D34.A 35.38,86.31 D33.A 35.43,83.55 D32.A 35.42,80.81 D31.A 35.43,78.13 D30.A 35.47,75.42 D29.A 35.5,72.63 D28.A 35.52,69.83 D27.A D26.A 35.53,64.34 D25.A 35.58,58.02 D1.A 35.55,55.14 D3.A 35.52,52.21 D2.A 35.48,49.09 D4.A 35.55,46.13 D5.A D6.A D7.A D8.A D9.A D10.A D11.A D12.A D13.A D14.A D15.A D16.A D17.A D18.A D19.A D20.A
  Top 0.813: U3.10 36.08,30.28 D11.A | 35.61,4.88 D20.A | 35.27,117.27 D48.A D47.A D42.A D46.A D45.A D44.A D43.A D41.A | U4.10 67.75,6 63.25,10.5 35.55,10.5 D18.A
  Top 1.27: 35.75,94.25 65.75,94.25 | 65.75,94.25 78.64,94.25 U1.16 | U5.4 72.55,121.05 66,114.5 66,110.25 | 66,110.25 66,94.5 65.75,94.25 | C1.+ 66.05,110.2 66,110.25
  Bottom 0.813: U3.10 75.21,28.5 82.12,28.5 87.71,22.91 U2.1 U2.24
A1_2  (via drill 0.5, 0.7)
  Top 0.305: J1.A12 14.02,49.3 14.02,48.84 16.05,46.81 v16.71,46.81 | J1.A1 13.7,55.16 14.94,56.4 v16.71,56.4 | D1.K v29.49,57.98 27.02,57.98 16.21,68.79 13.99,68.79 J3.7 | J5.5 9.32,82.18 10.38,81.12 10.38,72.38 8.5,70.5 8.5,69.03 J3.4
  Bottom 0.305: v16.71,46.81 v16.71,56.4 16.82,56.51 16.82,66.46 14.33,68.95 J3.7 13.8,68.92 10.92,68.92 9.84,67.83 J3.4 | 29.53,58.02 v29.49,57.98
  Bottom 0.406: R19.1 39.85,58.02 38.38,59.5 31.01,59.5 v29.49,57.98
B1_2  (via drill 0.5)
  Top 0.305: J1.B12 12.56,55.31 11.88,56 v11,56 12.68,57.68 20.43,57.68 22.97,55.14 v29.62,55.14 31.45,55.14 D3.K | J1.B1 12.56,49.51 v11.03,47.98
  Bottom 0.305: v11,56 10.55,56 8.85,54.3 8.85,50.15 v11.03,47.98 | 29.67,55.2 v29.62,55.14 30.98,56.5 38.25,56.5
  Bottom 0.406: R21.1 39.55,55.2 38.25,56.5
DN1  (via drill 0.5, 0.7)
  Top 0.254: J1.A7 16.68,51.8 16.69,51.81
  Top 0.305: v29.11,35.19 31.46,35.19 D9.K | 16.69,51.81 16.95,51.81 17.19,51.57 17.19,50.84 21.62,46.41 21.62,44.07 | 29.02,35.09 v29.11,35.19 | v29.11,35.19 26.05,38.25 25.96,38.25 21.62,42.59 21.62,44.07 | v22.61,44.07 21.62,44.07 | J3.2 11.75,70.28 11.75,82.62 10.25,84.13 J5.2
  Bottom 0.305: v22.61,44.07 5.14,44.07 4.28,44.93 4.28,68.06 5.26,69.04 10.18,69.04 11.34,70.2 J3.2 | R7.1 40.11,31.52 37.75,33.88 30.43,33.88 v29.11,35.19
DP1  (via drill 0.5, 0.7)
  Top 0.305: J1.A6 17.45,52.3 17.93,51.82 17.93,51.08 23.71,45.3 v23.71,43.09 23.71,42.96 28.63,38.04 v29.25,38.04 31.41,38.04 D8.K | J5.3 9.77,83.48 11,82.25 11,71.36 J3.3
  Bottom 0.305: J3.3 4.58,70.2 3.66,69.29 3.66,44.81 5.02,43.46 21.5,43.46 21.87,43.09 v23.71,43.09 | R6.1 40.8,33.83 38,36.62 30.67,36.62 v29.25,38.04
GND
  Top 1.27: C1.- 78,103.91 | 78,103.91 82.16,103.91 C2.- 95.75,104 SW4.B1 105.54,113.78 SW4.B | U5.1 77.69,104.22 78,103.91
  Bottom 0.61: U3.9 82.84,30.28 86.38,26.75 90.88,26.75 92.12,25.5 103.66,25.5 U2.23
  Bottom 0.813: R22.2 R27.2 43.55,52.1 R20.2 43.51,55.16 R21.2 43.47,57.97 R19.2 43.52,61.38 R23.2 48.57,61.44 SW2.3 SW2.4 | U4.9 94.87,6 108.38,19.5 108.38,23.75 106.75,25.38 103.78,25.38 U2.23 | BT1.1- 75.08,68.8 83.12,60.75 83.25,60.75 83.62,60.38 83.62,50.75 | 83.62,50.75 83.62,31.07 82.84,30.28 | U2.12 83.73,50.85 83.62,50.75
  Bottom 1.27: BT1.1- 68.82,68.8 SW2.4 | 75.08,68.8 75.08,71.7 U1.8 | SW2.3 55.5,75.61 55.5,83.25 | SW1.4 SW1.3 55.74,83.49 55.5,83.25 | 55.5,83.25 55.5,99.5 60,104 95.76,104 SW4.B1
  pour Bottom (isolate 0.813): 39.5,152.5 39.5,43 110.5,43 110.5,153 39.5,153
N$1
  Top 0.61: U2.2 94.2,25.45 99.25,30.5 99.25,77.25 89.38,87.12 83.22,87.12 U1.15
N$2
  Bottom 0.61: U2.3 89.87,27.99 92.38,30.5 92.38,58 80.12,70.25 80.12,86.38 76.62,89.88 75.47,89.88 U1.1
N$3
  Bottom 0.61: U2.21 100.22,30.53 94.75,36 94.75,59.25 85.5,68.5 85.5,73.38 84.38,74.5 83.15,74.5 U1.10
N$4
  Bottom 0.61: U2.22 100.76,27.99 93.62,35.12 93.62,58.62 83.25,69 83.25,71.86 U1.9
N$5
  Bottom 0.61: U3.18 57.1,50.6 47.25,40.75 43.76,40.75 R3.2
N$6
  Bottom 0.61: U3.17 56.06,48.06 46.25,38.25 43.79,38.25 R4.2
N$7
  Top 0.406: SW2.1 SW2.2 65.63,78.13 67.25,79.75 69.25,79.75 | 69.25,79.75 75.36,79.75 U1.5 | R1.1 69.17,79.83 69.25,79.75
N$8
  Top 0.406: U4.7 80.42,11.08 77.12,14.38 77.12,46.75 79.75,49.38 84.25,49.38 87.88,45.75 88.44,45.75 U2.10 88.49,45.75 89.62,45.75 90.75,44.62 90.75,42.75 90,42 87.12,42 83.6,45.52 U3.3
N$9
  Top 0.406: R2.1 72.17,83.05 73,82.22 U1.4
  Bottom 0.406: U1.4 72.92,82.22 SW1.2
  Bottom 0.61: SW1.1 SW1.2
N$10
  Top 0.406: U4.8 80.34,8.54 76.38,12.5 76.38,48.62 80,52.25 90.12,52.25 91.5,50.88 91.5,41.88 90.38,40.75 88.52,40.75 U2.8 86.81,40.69 84.38,43.12 81.19,43.12 U3.4
N$11
  Top 0.406: U2.7 87.35,38.15 85,40.5 81.11,40.5 U3.5
N$12
  Top 0.406: U2.6 88.14,35.61 85.88,37.88 81.08,37.88 U3.6
N$13
  Top 0.406: U2.5 87.93,33.07 85.75,35.25 81.16,35.25 U3.7
N$14
  Top 0.406: U2.4 88.09,30.53 85.88,32.75 81.12,32.75 U3.8
N$15
  Top 0.406: U4.4 106.57,18.7 109.62,21.75 109.62,32 106.12,35.5 103.82,35.5 U2.19
N$16
  Top 0.406: U4.1 81.56,26.32 86.88,21 98.75,21 101.38,23.62 101.38,36.5 103,38.12 103.68,38.12 U2.18
N$17
  Top 0.406: U4.2 79.85,23.78 78.75,24.88 78.75,27 80.12,28.38 81.88,28.38 86.12,24.12 98.38,24.12 100.5,26.25 100.5,38.12 103,40.62 103.64,40.62 U2.17
N$18
  Top 0.406: U4.3 82.26,21.24 83.75,19.75 105.88,19.75 108.38,22.25 108.38,31.62 107,33 103.78,33 U2.20
N$19  (via drill 0.5)
  Top 0.406: U4.5 81.97,16.16 83.5,14.62 83.5,8 82.75,7.25 79.88,7.25 75.62,11.5 v75.62,52.75 | U2.11 86.56,48.31 84.25,50.62 81.07,50.62 U3.1
  Bottom 0.406: v75.62,52.75 77.88,50.5 80.95,50.5 U3.1
N$20
  Top 0.406: U4.6 81.04,13.75 79.5,13.75 77.75,15.5 77.75,44.76 U3.2 81.11,48 83.12,48 87.89,43.23 U2.9
N$21
  Bottom 0.61: U3.16 55.27,45.52 46,36.25 43.86,36.25 R5.2
N$22
  Bottom 0.61: U3.15 54.48,42.98 45.5,34 43.92,34 R6.2
N$23
  Bottom 0.61: U3.14 54.19,40.44 45.25,31.5 43.76,31.5 R7.2
N$24
  Bottom 0.61: U3.13 53.65,37.9 45,29.25 43.82,29.25 R8.2
N$25
  Bottom 0.61: U3.12 53.86,35.36 45.5,27 R9.2
N$26
  Bottom 0.61: U3.11 53.32,32.82 45.25,24.75 43.83,24.75 R10.2
N$27
  Bottom 0.61: U4.18 49.32,26.32 45.5,22.5 43.89,22.5 R11.2
N$28
  Bottom 0.61: U4.17 48.78,23.78 45.5,20.5 43.8,20.5 R12.2
N$29
  Bottom 0.61: U4.16 48.74,21.24 45.75,18.25 43.86,18.25 R13.2
N$30
  Bottom 0.61: U4.15 48.7,18.7 45.75,15.75 43.83,15.75 R14.2
N$31
  Bottom 0.61: U4.14 48.16,16.16 45.5,13.5 43.77,13.5 R15.2
N$32
  Bottom 0.61: U4.13 47.87,13.62 45.5,11.25 43.83,11.25 R16.2
N$33
  Bottom 0.61: U4.12 48.08,11.08 46,9 43.76,9 R17.2
N$34
  Bottom 0.61: U4.11 48.04,8.54 46.25,6.75 43.83,6.75 R18.2
N$35
  Top 0.61: J5.SH5 4.54,81.33 J5.SH4 J5.SH3 3.54,86.08 J5.SH1
  Bottom 0.305: R24.1 36.5,65 35.88,65.62 27.5,65.62 13.25,79.88
  Bottom 0.406: 13.25,79.88 J5.SH6 J5.SH5 | J5.SH2 J5.SH1
N$36
  Top 0.406: J6.1 9.41,122.91 10.75,124.25 10.75,135.42 J4.1 10.28,136.12 23,136.12 30.35,128.78 D42.K
N$37
  Top 0.305: 3.32,107.74 0.79,105.21 0.79,96.59 6.08,91.3 7.48,91.3 14.24,84.54 14.24,79.86 29.82,64.29 D25.K | 3.32,107.74 3.37,107.79 | J2.B11 3.32,107.74
N$38  (via drill 0.7)
  Top 0.254: J1.A5 17.81,52.8 18.42,52.19 18.42,51.45 28.26,41.61
  Top 0.305: D7.K 29.88,40.71 29.82,40.66 29.21,40.66 v29.2,40.67 | 29.15,40.63 v29.2,40.67 | 28.02,41.86 28.26,41.61 v29.2,40.67
  Bottom 0.305: R5.1 39.74,36.14 36.62,39.25 36.5,39.25 36.38,39.38 30.5,39.38 v29.2,40.67
N$39  (via drill 0.5)
  Top 0.406: J6.2 13.14,122.26 14.5,123.62 v18.38,123.62 | D43.K 29.47,140.03 26.12,143.38 10,143.38 6.12,139.5 6.12,138 6.88,137.25 8.91,137.25 J4.2
  Bottom 0.406: v18.38,123.62 18.38,138.25 13.75,142.88 9.5,142.88 6.12,139.5 6.12,138 6.75,137.38 8.88,137.38 10.01,138.51 J4.2
N$40  (via drill 0.5)
  Top 0.406: J6.3 16.49,121.61 v16.62,121.75 | J4.3 8.25,138.59 8.25,140.25 10.5,142.5 22.88,142.5 28.12,137.25 31.21,137.25 D44.K
  Bottom 0.406: v16.62,121.75 16.62,135.75 14,138.38 12,138.38 10.5,139.88 9.53,139.88 J4.3
N$41  (via drill 0.7)
  Top 0.254: J1.A8 14.76,51.3 14.81,51.36 14.84,51.36 14.89,51.41 16.4,51.41 16.56,51.25
  Top 0.305: v28.84,32.46 D10.K | 16.56,51.25 16.56,50.48 20.76,46.28 20.76,40.5 25.27,35.99 25.31,35.99 v28.84,32.46 | 28.76,32.39 v28.84,32.46
  Bottom 0.305: R8.1 39.93,29.32 38.12,31.12 30.18,31.12 v28.84,32.46
N$42
  Top 0.406: D45.K 29.1,134.4 22,141.5 J4.5
N$43
  Top 0.406: D46.K 30.35,131.53 22.12,139.75 J4.6
N$44
  Top 0.305: J2.B10 3.84,107.24 1.37,104.76 1.37,97.08 6.53,91.92 7.84,91.92 14.98,84.78 14.98,80.6 28.45,67.13 D26.K
N$45  (via drill 0.7)
  Top 0.254: 11.41,49.4 12.07,50.05
  Top 0.305: J1.B2 12.07,50.05 | 11.41,49.4 5.55,49.4 5.03,48.88 5.03,29.18 9.94,24.27 28.62,24.27 28.66,24.23 v29.34,24.23 31.48,24.23 D13.K
  Bottom 0.305: R11.1 39.36,22.64 39.12,22.88 30.69,22.88 v29.34,24.23
N$46  (via drill 0.7)
  Top 0.305: J1.B3 11.85,50.55 11.16,49.86 5.14,49.86 4.51,49.24 4.51,28.09 11.29,21.32 29.67,21.32 v29.73,21.38 31.4,21.38 D14.K
  Bottom 0.305: R12.1 39.45,20.45 39.12,20.12 30.98,20.12 v29.73,21.38
N$47  (via drill 0.7)
  Top 0.305: J1.B5 11.64,51.55 11.54,51.45 5.7,51.45 4.04,49.79 4.04,27.34 13.01,18.36 29.78,18.36 v29.79,18.38 31.11,18.34 D15.K
  Bottom 0.305: R13.1 39.39,18.14 38.62,17.38 30.79,17.38 v29.79,18.38
N$48  (via drill 0.7)
  Top 0.305: J1.B6 11.53,52.05 11.46,51.99 11.44,51.99 11.39,51.94 5.53,51.94 3.52,49.94 3.52,26.74 14.36,15.9 29.86,15.9 v29.9,15.86 31.39,15.86 D16.K
  Bottom 0.305: 29.93,15.83 v29.9,15.86 31.14,14.62 38,14.62 39.2,15.83 R14.1
N$49  (via drill 0.7)
  Top 0.305: J1.B7 11.4,52.55 11.31,52.46 11.3,52.46 11.28,52.44 5.36,52.44 3.02,50.1 3.02,25.89 15.59,13.32 29.91,13.32 v30.01,13.21 D17.K
  Bottom 0.305: R15.1 38.83,13.48 38.55,13.2 38.55,13.05 37.38,11.88 31.35,11.88 v30.01,13.21 30.3,13.2
N$50  (via drill 0.7)
  Top 0.305: D18.K 30.86,10.46 | 30.86,10.46 v29.94,10.46 | J1.B8 11.05,53.05 10.91,52.91 5.04,52.91 2.5,50.38 2.5,25.18 17.19,10.49 29.91,10.49 v29.94,10.46 | v29.94,10.46 30.86,10.46
  Bottom 0.305: v29.94,10.46 30.5,10.46 31.84,9.12 37.88,9.12 39.92,11.17 R16.1
N$51  (via drill 0.7)
  Top 0.305: D19.K 30.94,7.71 | 30.94,7.71 v29.93,7.71 | J1.B10 11.53,54.05 11.07,54.51 5.76,54.51 2,50.75 2,24.45 18.79,7.66 29.88,7.66 v29.93,7.71 | v29.93,7.71 30.94,7.71
  Bottom 0.305: 29.96,7.75 v29.93,7.71 31.26,6.38 36.75,6.38 39.36,8.99 R17.1
N$52  (via drill 0.7)
  Top 0.305: v30,4.96 D20.K v30,4.96 | J1.B11 12.54,54.58 11.76,54.58 11.72,54.61 11.72,54.84 11.49,55.08 5.56,55.08 5.44,54.95 5.44,54.94 1.38,50.88 1.38,23.73 20.27,4.83 29.87,4.83 v30,4.96
  Bottom 0.305: R18.1 40.3,6.67 36.5,2.88 32.09,2.88 v30,4.96 30.04,4.92
N$53
  Top 0.305: J2.B8 7.89,106.24 7.42,105.76 7.39,105.76 7.23,105.6 3.09,105.6 1.88,104.39 1.88,97.7 3.48,96.1 4.4,96.1 7.72,92.78 7.84,92.78 15.84,84.78 15.84,80.85 26.88,69.81 D27.K
N$54
  Top 0.305: J2.B7 8.04,105.74 7.5,105.2 7.49,105.2 7.45,105.16 3.44,105.16 2.43,104.15 2.43,98.07 3.78,96.72 4.89,96.72 16.58,85.03 16.58,81.09 25.06,72.61 D28.K
N$55
  Top 0.305: J2.B6 8.23,105.24 7.73,104.74 7.73,104.72 7.69,104.69 4.29,104.69 4.28,104.67 3.69,104.67 3,103.99 3,98.56 4.11,97.45 5.14,97.45 17.44,85.15 17.44,81.46 23.53,75.38 D29.K
N$56
  Top 0.305: J2.B5 8.44,104.74 7.97,104.26 7.94,104.26 7.9,104.22 4.12,104.22 3.54,103.65 3.54,99.17 4.65,98.07 5.63,98.07 18.18,85.52 18.18,81.71 21.8,78.09 D30.K
N$57
  Top 0.305: J2.B3 8.82,103.74 8.33,103.25 5.63,103.25 4.12,101.74 4.12,99.94 5.25,98.81 6,98.81 24.02,80.79 D31.K
N$58
  Top 0.305: 11.41,103.24 J2.B2 9.01,103.24 8.52,102.75 6.03,102.75 4.77,101.49 4.77,100.57 5.67,99.67 6.12,99.67 22.26,83.53 D32.K
N$59
  Top 0.254: 17.56,101.51 15.38,101.51 15.34,101.47
  Top 0.305: 15.34,101.47 13.83,102.99 J2.A11 | D33.K 30.35,86.25 28.02,88.59 28.02,91.06 17.56,101.51
N$60
  Top 0.305: J2.A10 14.23,103.49 15.7,102.01 18.05,102.01 19.04,101.03 19.04,101.02 29,91.06 29,90.46 30.48,88.99 D34.K
N$61
  Top 0.305: J2.A8 16.58,104.49 19.78,101.29 19.78,101.27 29,92.04 29,91.94 29.62,91.33 30.99,91.33 D35.K
N$62
  Top 0.305: J2.A7 16.94,104.99 | 16.94,104.99 | 16.94,104.99 17.07,104.99 20.39,101.67 20.39,101.64 27.4,94.62 31.13,94.62 D36.K
N$63
  Top 0.305: J2.A6 16.91,105.49 | 16.91,105.49 16.92,105.49 | D37.K 25.8,97.1 17.41,105.49 16.91,105.49
N$64
  Top 0.305: J2.A5 17.88,105.99 24.08,99.79 31.27,99.79 D38.K 31.1,99.76
N$65
  Top 0.305: J2.A3 14.53,106.99 15.4,107.86 17.32,107.86 17.32,107.78 22.85,102.25 31.13,102.25 D39.K 31.18,102.3 30.71,102.3
N$66
  Top 0.305: J2.A2 14.09,107.49 14.93,108.32 17.64,108.32 20.88,105.08 30.71,105.08 30.72,105.09 | 30.05,105.09 30.72,105.09 | 30.72,105.09 31.26,105.09 D40.K
N$67
  Top 0.406: J3.SH2 J3.SH1
  Bottom 0.406: R23.1 29.81,61.44 15.62,75.62 7.78,75.62 J3.SH1
N$68
  Top 0.406: D47.K 30.22,125.9 21.38,134.75 J4.8
N$69
  Top 0.406: D48.K 30.35,123.15 20.62,132.88 12.29,132.88 J4.9
N$75
  Top 0.61: J1.SH4 8.76,47.87 9.75,46.88 12.24,46.88 J1.SH2
  Bottom 0.305: 28.84,50.23 28.85,50.23 29.25,50.62 36.86,50.62 R27.1
  Bottom 0.406: 28.84,50.23 24.41,45.8 24.36,45.8 24.23,45.66 15.44,45.66 J1.SH2
  Bottom 0.61: J1.SH3 9.43,57.25 12.5,57.25 J1.SH1 J1.SH2
N$120
  Top 1.27: BT1.2+ 90.55,141.7 93.75,138.5 93.75,118.25 95.75,116.25 100.2,116.25 SW4.2
N$121
  Top 1.27: C2.+ U5.3 82.5,113.61 SW4.3
N$122
  Bottom 1.27: BT1.2- 96.8,68.8 108.75,80.75 108.75,125.25 105.75,128.25 83.25,128.25 69.8,141.7 BT1.1+
RX2+  (via drill 0.5, 0.7)
  Top 0.254: J1.A11 14.21,49.8 14.82,49.19 14.82,48.9
  Top 0.305: v29.34,26.95 31.48,26.95 D12.K | 29.27,27.01 v29.34,26.95 | 14.82,48.9 15.96,47.76 17.56,47.76 18.42,46.9 v18.42,42.59 18.42,37.86 v29.34,26.95
  Bottom 0.305: J3.6 4.72,71.45 3.05,69.78 3.05,44.19 4.65,42.59 v18.42,42.59 | R10.1 39.17,24.83 38.38,25.62 30.66,25.62 v29.34,26.95
RX2-  (via drill 0.5, 0.7)
  Top 0.254: J1.A10 14.36,50.3 15.16,49.5 15.21,49.5 16.33,48.38
  Top 0.305: v29.04,29.77 31.43,29.77 D11.K | 16.33,48.38 17.81,48.38 19.65,46.53 v19.65,41.73 19.65,39.16 v29.04,29.77 | 28.94,29.68 v29.04,29.77
  Bottom 0.305: J3.5 12.99,73.2 12.03,72.24 4.65,72.24 2.43,70.02 2.43,43.58 4.28,41.73 v19.65,41.73 | R9.1 39.74,27.01 38.5,28.25 38.38,28.25 38.25,28.38 30.44,28.38 v29.04,29.77
SHIELD
  Top 0.61: D41.K 29.72,142.78 27.88,144.62 6.8,144.62 J4.SH1 | J2.SH1 J2.SH3 | J2.SH4 J2.SH2
  Bottom 0.61: J4.SH2 4.86,131.24 2.25,128.62 2.25,115.63 J2.SH3 | J2.SH2 J2.SH1
  Bottom 0.813: J4.SH1 5.45,142.08 4.62,141.25 4.62,132.06 J4.SH2
TX1+  (via drill 0.5, 0.7)
  Top 0.254: J1.A2 14.37,54.3 14.68,54.61 14.68,54.8 14.99,55.11 15,55.11 15.11,55.23 v20.09,55.23 | 20.34,54.97 v29.5,45.81
  Top 0.305: J3.9 15.38,64.7 16.33,63.75 19.78,63.75 v19.9,63.87 | v20.09,55.23 20.34,54.97
  Top 0.406: v29.5,45.81 31.45,45.81 D5.K
  Bottom 0.305: v19.9,63.87 19.9,55.41 v20.09,55.23 | v29.5,45.81 29.5,45.62 30.5,44.62 35.88,44.62 39.75,40.75 40.89,40.75 R3.1
  Bottom 0.406: 29.58,45.89 v29.5,45.81
TX1-  (via drill 0.5, 0.7)
  Top 0.254: J1.A3 14.53,53.8 15.3,54.58 15.36,54.58 15.38,54.59 18.23,54.59 v18.79,54.03 | 19.15,53.66 v29.5,43.31
  Top 0.305: D6.K v29.5,43.31 | J3.8 16.59,66.45 v18.3,64.73 | v18.79,54.03 19.15,53.66
  Bottom 0.305: 29.52,43.33 v29.5,43.31 30.81,42 35.62,42 39.42,38.21 R4.1 | v18.3,64.73 18.3,54.51 v18.79,54.03
VBUS_A  (via drill 0.5, 0.7)
  Top 0.254: v15.66,53.79 17.56,53.79 v19.16,52.19
  Top 0.305: J1.A4 14.94,53.3 v15.66,53.79 | J1.A9 13.71,50.81 15.25,50.81 v15.62,50.44 | D2.K 29.52,52.17 v29.49,52.14 | J3.1 11.84,68.46 13.38,70 14.5,70 15.62,71.12 15.62,74.38 12.88,77.12 12.88,82.25 10.35,84.78 J5.1
  Bottom 0.254: v19.16,52.19 25.56,52.19
  Bottom 0.305: v15.62,50.44 15.62,53.75 v15.66,53.79 15.66,66.51 14.49,67.69 11.85,67.69 J3.1 | 25.56,52.19 25.6,52.14 v29.49,52.14 30.98,53.62 38.12,53.62 39.61,52.14 R20.1
VBUS_B  (via drill 0.5, 0.7)
  Top 0.305: J1.B9 10.64,53.55 v10.45,53.75 | J1.B4 11.78,51.05 11.68,50.95 10.24,50.95 v9.95,50.66 | v29.49,48.98 31.49,48.98 D4.K
  Bottom 0.305: v10.45,53.75 9.95,53.25 v9.95,50.66 12.06,48.55 12.06,47.11 14.22,44.95 25.11,44.95 29.18,49.01 29.45,49.01 v29.49,48.98 29.49,48.51 30.38,47.62 30.5,47.62 30.62,47.5 35.75,47.5 40.12,43.12 40.7,43.12 R22.1

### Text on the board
tPlace: SHIELD | DN | DP | SSRX- | USB 3 | SSRX+ | VBUS | SSTX- | SSTX+ | VBUS B | USB 2 MICRO | GND B | VBUS A | GND A | GND A | TX1+ | TX1- | TYPE C | CC1 | DN1 | DP1 | A2 | SBU1 | RX2- | RX2+ | TX2+ | DOWN | TX2- | USB 2 MICRO | CC2 | DN2 | B2 | UP | DP2 | SBU2 | RX- | USB 3 | RX+ | GND A | RADIOSCH.EU | GND B | VBUS A | VBUS B | TYPE C | TX1+ | TX1- | CC1 | DN1 | A1 | A1 | DP1 | SBU1 | RX2- | RX2+ | TX2+ | TX2- | CC2 | DP2 | B1 | DN2 | SBU2 | RX1- | RX1+
bPlace: RADIOSCH.EU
